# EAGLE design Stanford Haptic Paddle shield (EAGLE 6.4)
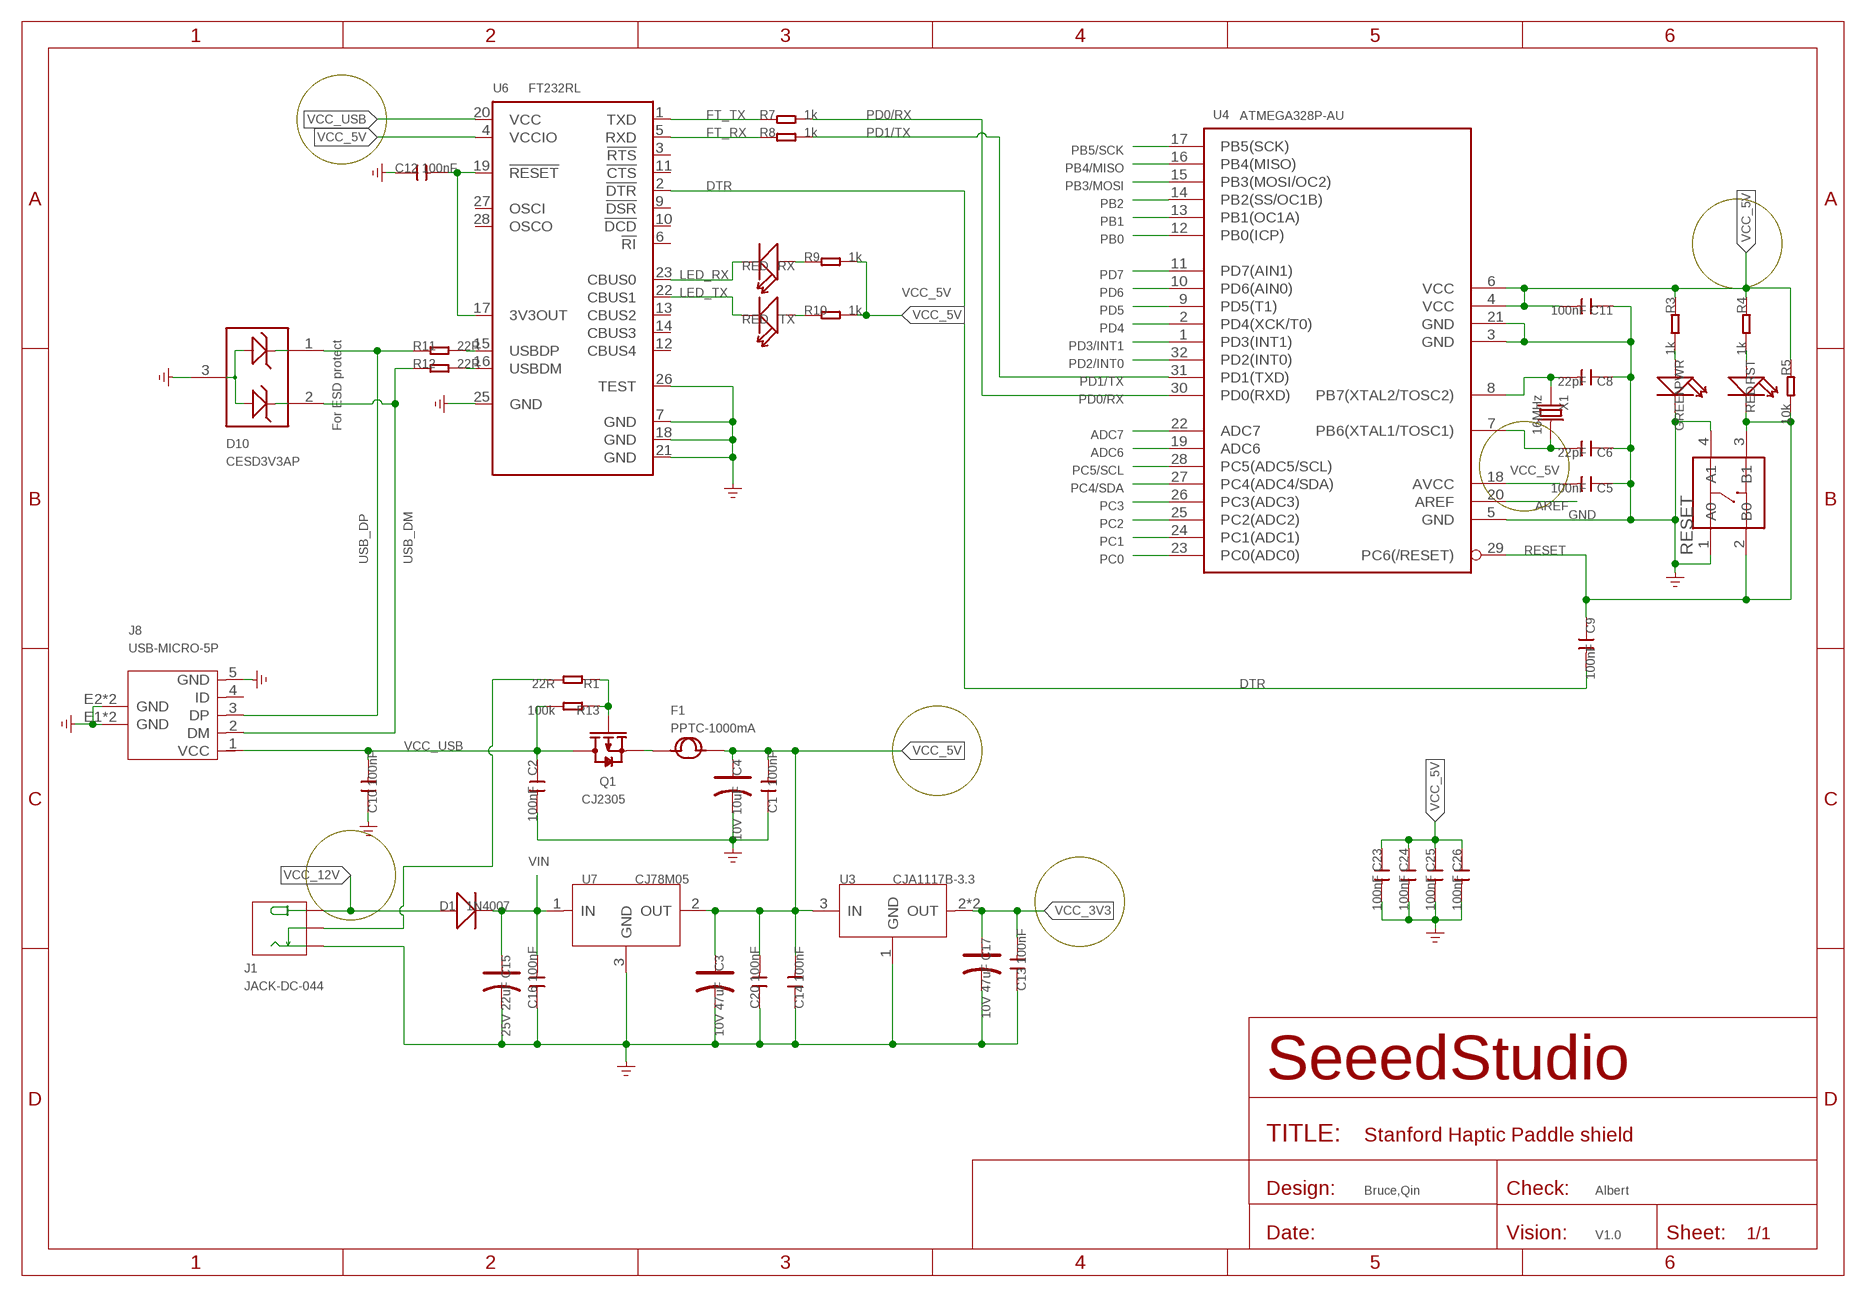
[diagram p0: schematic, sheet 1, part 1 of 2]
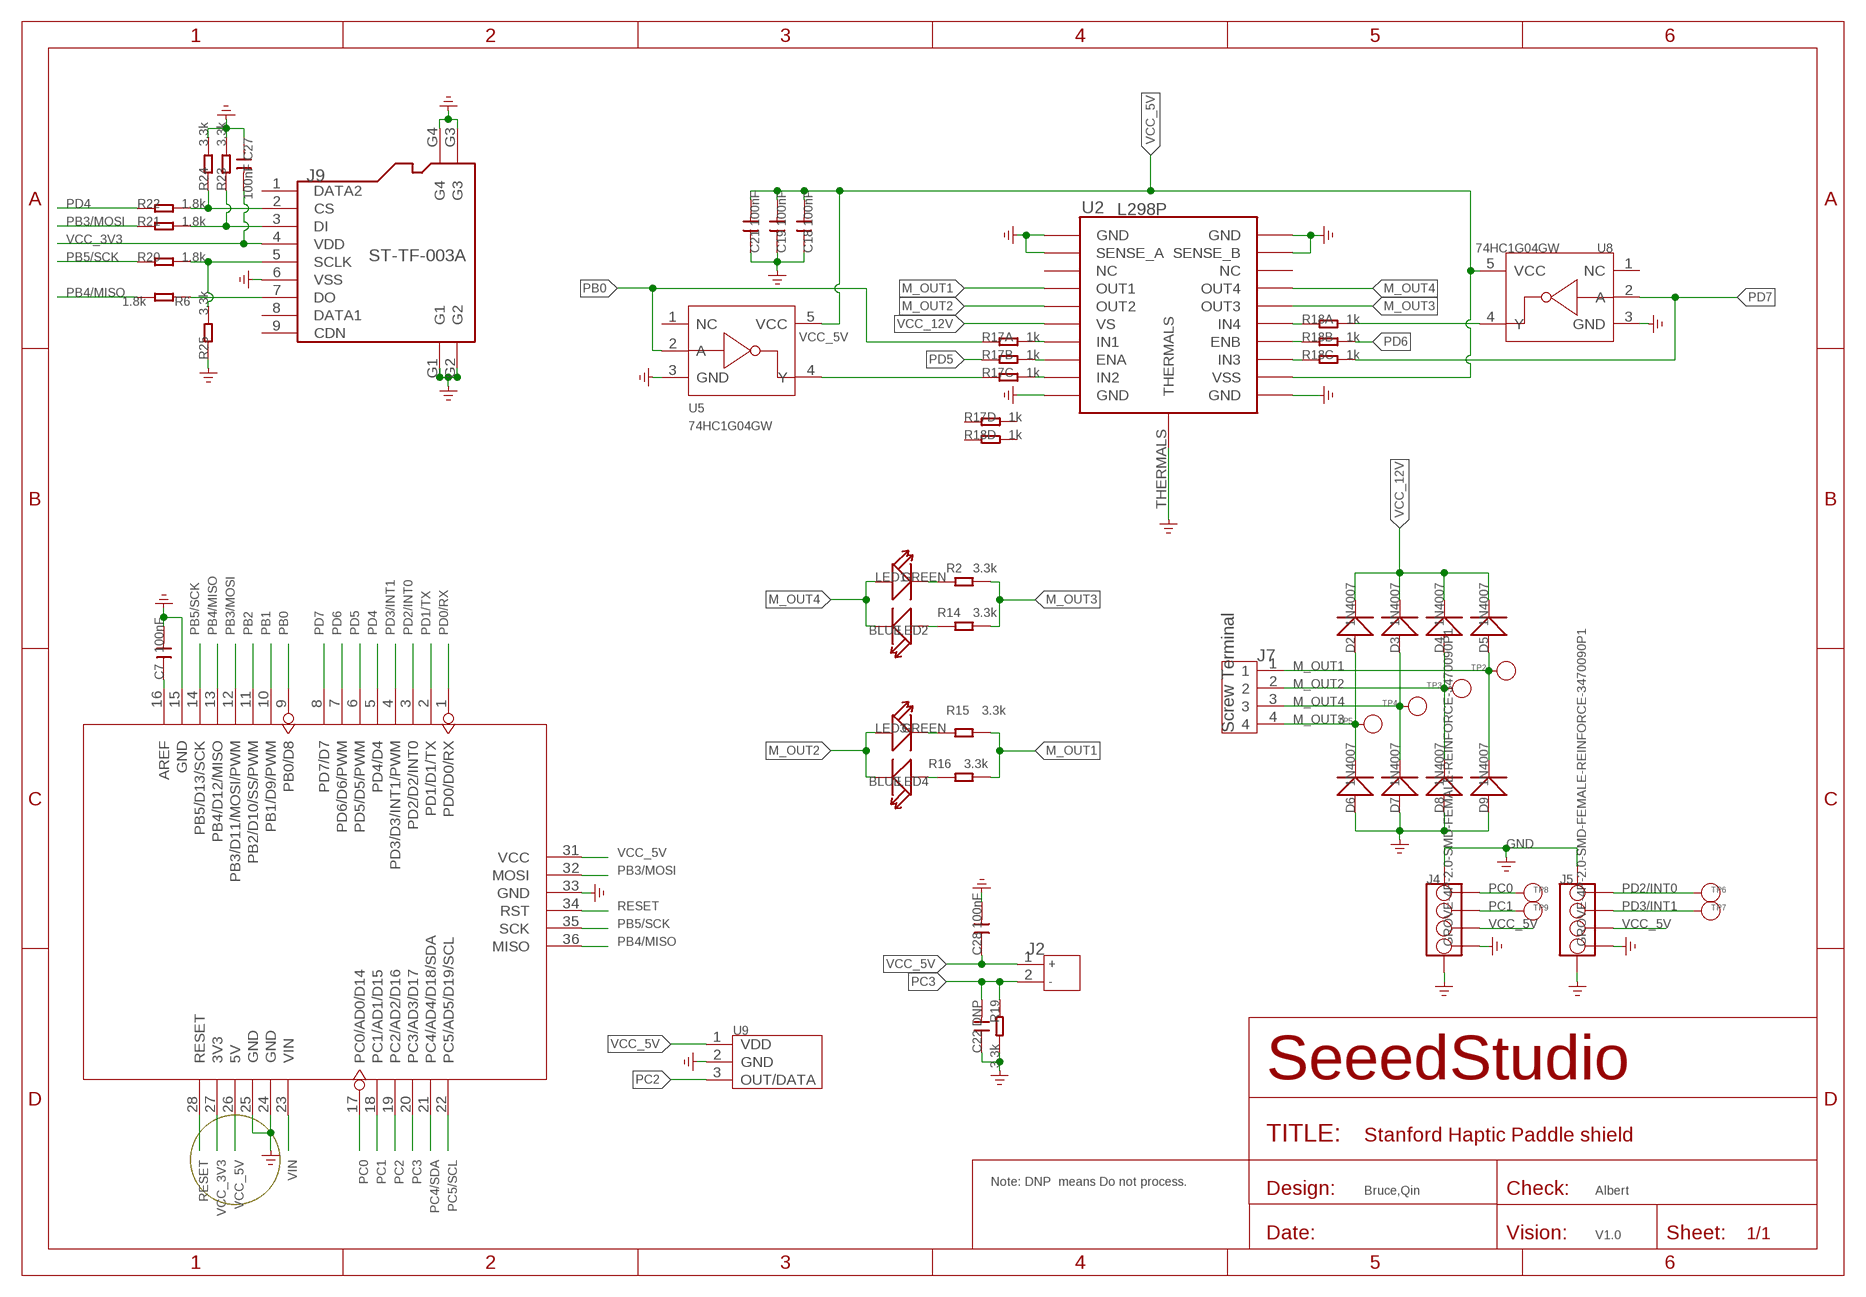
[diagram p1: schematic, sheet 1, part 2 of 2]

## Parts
C1  100nF  C-0603  [C0603]
C2  100nF  C-0603  [C0603]
C3  10V 47uF  CAP-AVX-B  [AVX-B]
C4  10V 10uF  C-POLAR-A  [AVX-A]
C5  100nF  C-0603  [C0603]
C6  22pF  C-0603  [C0603]
C7  100nF  C-0603  [C0603]
C8  22pF  C-0603  [C0603]
C9  100nF  C-0603  [C0603]
C10  100nF  C-0603  [C0603]
C11  100nF  C-0603  [C0603]
C12  100nF  C-0603  [C0603]
C13  100nF  C-0603  [C0603]
C14  100nF  C-0603  [C0603]
C15  25V 22uF  C-POLAR-C  [AVX-C]
C16  100nF  C-0603  [C0603]
C17  10V 47uF  CAP-AVX-B  [AVX-B]
C18  100nF  C-0603  [C0603]
C19  100nF  C-0603  [C0603]
C20  100nF  C-0603  [C0603]
C21  100nF  C-0603  [C0603]
C22  DNP  C-0603  [C0603]
C23  100nF  C-0603  [C0603]
C24  100nF  C-0603  [C0603]
C25  100nF  C-0603  [C0603]
C26  100nF  C-0603  [C0603]
C27  100nF  C-0603  [C0603]
C28  100nF  C-0603  [C0603]
D1  1N4007  D'B130L-13-F'  [SMA]
D2  1N4007  D'B130L-13-F'  [SMA]
D3  1N4007  D'B130L-13-F'  [SMA]
D4  1N4007  D'B130L-13-F'  [SMA]
D5  1N4007  D'B130L-13-F'  [SMA]
D6  1N4007  D'B130L-13-F'  [SMA]
D7  1N4007  D'B130L-13-F'  [SMA]
D8  1N4007  D'B130L-13-F'  [SMA]
D9  1N4007  D'B130L-13-F'  [SMA]
D10  CESD3V3AP  D-ESD-3P  [SOT23]
F1  PPTC-1000mA  FUSE'1206'  [F1206]
J1  JACK-DC-044  [DC-044]
J2  JACK-JST-2P-PW'2.0'  [JST-2.0]
J4  GROVE-4P-2.0-SMD-FEMALE-REINFORCE-3470090P1  [4P-SMD-2.0]
J5  GROVE-4P-2.0-SMD-FEMALE-REINFORCE-3470090P1  [4P-SMD-2.0]
J7  Screw Terminal  SCREW-TERMINAL-4P'3.5'  [4P-3.5]
J8  USB-MICRO-5P  [MICRO-USB-5P]
J9  ST-TF-003A  HOLDER-MICROSD-9P  [9P-SMD-W/-RING]
LED1  GREEN  LED'0603'  [LED-0603]
LED2  BLUE  LED'0603'  [LED-0603]
LED3  GREEN  LED'0603'  [LED-0603]
LED4  BLUE  LED'0603'  [LED-0603]
PWR  GREEN  LED'0603'  [LED-0603]
Q1  CJ2305  MOSFET-P'SI2323CDS/SI2305DS<BR>'  [SOT23]
R1  22R  R-0603  [R0603]
R2  3.3k  R-0603  [R0603]
R3  1k  R-0603  [R0603]
R4  1k  R-0603  [R0603]
R5  10k  R-0603  [R0603]
R6  1.8k  R-0603  [R0603]
R7  1k  R-0603  [R0603]
R8  1k  R-0603  [R0603]
R9  1k  R-0603  [R0603]
R10  1k  R-0603  [R0603]
R11  22R  R-0603  [R0603]
R12  22R  R-0603  [R0603]
R13  100k  R-0603  [R0603]
R14  3.3k  R-0603  [R0603]
R15  3.3k  R-0603  [R0603]
R16  3.3k  R-0603  [R0603]
R17  1k  R-4R-1206  [1206-8-3.3X2.4]
R18  1k  R-4R-1206  [1206-8-3.3X2.4]
R19  3.3k  R-0603  [R0603]
R20  1.8k  R-0603  [R0603]
R21  1.8k  R-0603  [R0603]
R22  1.8k  R-0603  [R0603]
R23  3.3k  R-0603  [R0603]
R24  3.3k  R-0603  [R0603]
R25  3.3k  R-0603  [R0603]
RESET  BUTTON-4P-6X6-SMD  [4P-SMD-6.2X6.2X4H]
RST  RED  LED'0603'  [LED-0603]
RX  RED  LED'0603'  [LED-0603]
TP2  PAD-TEST-POINT'3535'  [TP_3535]
TP3  PAD-TEST-POINT'3535'  [TP_3535]
TP4  PAD-TEST-POINT'3535'  [TP_3535]
TP5  PAD-TEST-POINT'3535'  [TP_3535]
TP6  PAD-TEST-POINT'3535'  [TP_3535]
TP7  PAD-TEST-POINT'3535'  [TP_3535]
TP8  PAD-TEST-POINT'3535'  [TP_3535]
TP9  PAD-TEST-POINT'3535'  [TP_3535]
TX  RED  LED'0603'  [LED-0603]
U1  ARDUINO'W/O-SILK'  [ARDUINO-W/O-SILK]
U2  L298P  [POWERSO-20]
U3  CJA1117B-3.3  CJ1117-3.3-1310120P1  [SOT89]
U4  ATMEGA328P-AU  ATMEGA8/168/328  [TQFP32]
U5  74HC1G04GW  74HC1G04  [SOT-353]
U6  FT232RL  [SSOP28]
U7  CJ78M05  78M05-TO252  [TO252]
U8  74HC1G04GW  74HC1G04  [SOT-353]
U9  SENSOR-MR-KMA210  [3P-5.55X1.55]
X1  16MHz  CRYSTAL'5032'  [2P-SMD-5X3.2]

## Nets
ADC6: U4.19(ADC6)
ADC7: U4.22(ADC7)
AREF: C7.1 U1.16(AREF) U4.20(AREF)
DTR: C9.2 U6.2(!DTR)
FT_RX: R8.1 U6.5(RXD)
FT_TX: R7.1 U6.1(TXD)
GATE: J1.CDN R1.2
GND: C1.1 C2.2 C3.- C4.- C5.1 C6.1 C7.2 C8.1 C10.1 C11.1 C12.1 C13.1 C14.1 C15.- C16.1 C17.- C18.1 C19.1 C20.1 C21.1 C22.1 C23.2 C24.2 C25.2 C26.2 C27.1 C28.2 D6.2(+) D7.2(+) D8.2(+) D9.2(+) D10.3 J1.- J4.4 J4.SS1 J4.SS2 J5.4 J5.SS1 J5.SS2 J8.5(GND) J8.E1(GND) J8.E2(GND) J8.P1(GND) J8.P2(GND) J9.6(VSS) J9.G1 J9.G2 J9.G3 J9.G4 PWR.- R19.2 R23.2 R24.2 R25.1 RESET.1(A0) RESET.4(A1) U1.15(GND) U1.24(GND) U1.25(GND) U1.33(GND) U2.P$1(GND) U2.P$2(SENSE_A) U2.P$10(GND) U2.P$11(GND) U2.P$19(SENSE_B) U2.P$20(GND) U2.THERMALS U3.1(GND) U4.3(GND) U4.5(GND) U4.21(GND) U5.3(GND) U6.7(GND) U6.18(GND) U6.21(GND) U6.25(GND) U6.26(TEST) U7.3(GND) U8.3(GND) U9.2(GND)
LED_RX: RX.- U6.23(CBUS0)
LED_TX: TX.- U6.22(CBUS1)
M_IN2: R17.3 U5.4(Y)
M_IN4: R18.8 U8.4(Y)
M_OUT1: D5.2(+) D9.1(-) J7.1 R15.1 R16.1 TP2.T U2.P$4(OUT1)
M_OUT2: D4.2(+) D8.1(-) J7.2 LED3.+ LED4.- TP3.T U2.P$5(OUT2)
M_OUT3: D2.2(+) D6.1(-) J7.4 R2.1 R14.1 TP5.T U2.P$16(OUT3)
M_OUT4: D3.2(+) D7.1(-) J7.3 LED1.+ LED2.- TP4.T U2.P$17(OUT4)
N$1: Q1.1(G) R1.1 R13.1
N$2: R12.2 U6.16(USBDM)
N$3: J9.7(DO) R6.1
N$4: R11.2 U6.15(USBDP)
N$5: LED1.- R2.2
N$6: C12.2 U6.17(3V3OUT) U6.19(!RESET)
N$7: PWR.+ R3.2
N$8: LED2.+ R14.2
N$9: LED3.- R15.2
N$10: LED4.+ R16.2
N$11: J9.5(SCLK) R20.2 R25.2
N$12: J9.3(DI) R21.2 R23.1
N$13: J9.2(CS) R22.2 R24.1
N$14: R17.8 U2.P$7(IN1)
N$15: R17.7 U2.P$8(ENA)
N$16: R17.6 U2.P$9(IN2)
N$17: R4.2 RST.+
N$21: R18.3 U2.P$13(IN3)
N$22: R18.2 U2.P$14(ENB)
N$23: R18.1 U2.P$15(IN4)
N$31: R9.1 RX.+
N$32: R10.1 TX.+
P5V: F1.1 Q1.2(S)
PB0: R17.1 U1.9(PB0/D8) U4.12(PB0(ICP)) U5.2(A)
PB1: U1.10(PB1/D9/PWM) U4.13(PB1(OC1A))
PB2: U1.11(PB2/D10/SS/PWM) U4.14(PB2(SS/OC1B))
PB3/MOSI: R21.1 U1.12(PB3/D11/MOSI/PWM) U1.32(MOSI) U4.15(PB3(MOSI/OC2))
PB4/MISO: R6.2 U1.13(PB4/D12/MISO) U1.36(MISO) U4.16(PB4(MISO))
PB5/SCK: R20.1 U1.14(PB5/D13/SCK) U1.35(SCK) U4.17(PB5(SCK))
PC0: J4.1 TP8.T U1.17(PC0/AD0/D14) U4.23(PC0(ADC0))
PC1: J4.2 TP9.T U1.18(PC1/AD1/D15) U4.24(PC1(ADC1))
PC2: U1.19(PC2/AD2/D16) U4.25(PC2(ADC2)) U9.3(OUT/DATA)
PC3: C22.2 J2.2 R19.1 U1.20(PC3/AD3/D17) U4.26(PC3(ADC3))
PC4/SDA: U1.21(PC4/AD4/D18/SDA) U4.27(PC4(ADC4/SDA))
PC5/SCL: U1.22(PC5/AD5/D19/SCL) U4.28(PC5(ADC5/SCL))
PD0/RX: R7.2 U1.1(PD0/D0/RX) U4.30(PD0(RXD))
PD1/TX: R8.2 U1.2(PD1/D1/TX) U4.31(PD1(TXD))
PD2/INT0: J5.1 TP6.T U1.3(PD2/D2/INT0) U4.32(PD2(INT0))
PD3/INT1: J5.2 TP7.T U1.4(PD3/D3/INT1/PWM) U4.1(PD3(INT1))
PD4: R22.1 U1.5(PD4/D4) U4.2(PD4(XCK/T0))
PD5: R17.2 U1.6(PD5/D5/PWM) U4.9(PD5(T1))
PD6: R18.7 U1.7(PD6/D6/PWM) U4.10(PD6(AIN0))
PD7: R18.6 U1.8(PD7/D7) U4.11(PD7(AIN1)) U8.2(A)
RESET: C9.1 R5.2 RESET.2(B0) RESET.3(B1) RST.- U1.28(RESET) U1.34(RST) U4.29(PC6(/RESET))
USB_DM: D10.2 J8.2(DM) R12.1
USB_DP: D10.1 J8.3(DP) R11.1
VCC_3V3: C13.2 C17.+ C27.2 J9.4(VDD) U1.27(3V3) U3.2(OUT) U3.4(OUT)
VCC_5V: C1.2 C3.+ C4.+ C5.2 C11.2 C14.2 C18.2 C19.2 C20.2 C21.2 C23.1 C24.1 C25.1 C26.1 C28.1 F1.2 J2.1 J4.3 J5.3 R3.1 R4.1 R5.1 R9.2 R10.2 U1.26(5V) U1.31(VCC) U2.P$12(VSS) U3.3(IN) U4.4(VCC) U4.6(VCC) U4.18(AVCC) U5.5(VCC) U6.4(VCCIO) U7.2(OUT) U8.5(VCC) U9.1(VDD)
VCC_12V: D1.2(+) D2.1(-) D3.1(-) D4.1(-) D5.1(-) J1.+ U2.P$6(VS)
VCC_USB: C2.1 C10.2 J8.1(VCC) Q1.3(D) R13.2 U6.20(VCC)
VIN: C15.+ C16.2 D1.1(-) U1.23(VIN) U7.1(IN)
XTAL1: C6.2 U4.7(PB6(XTAL1/TOSC1)) X1.2
XTAL2: C8.2 U4.8(PB7(XTAL2/TOSC2)) X1.1
Unconnected: J8.4(ID) J9.1(DATA2) J9.8(DATA1) J9.9(CDN) R17.4 R17.5 R18.4 R18.5 U2.P$3(NC) U2.P$18(NC) U5.1(NC) U6.3(!RTS) U6.6(!RI) U6.9(!DSR) U6.10(!DCD) U6.11(!CTS) U6.12(CBUS4) U6.13(CBUS2) U6.14(CBUS3) U6.27(OSCI) U6.28(OSCO) U8.1(NC)

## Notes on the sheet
- For ESD protect
- Note: DNP  means Do not process.
- Bruce,Qin | Albert | Bruce,Qin | Albert
- V1.0 | V1.0

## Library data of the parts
C1 C2 C5-C14 C16 C18-C28 = Discrete:C*: Ceramic Capacitors
C3 C17 = Discrete:CAP*: Electrolytic Capacitors,Tantalum Capacitors and Super Capacitors
C4 C15 = OPL:C-POLAR*
D1-D9 = Discrete:D*
D10 = Discrete:D-ESD-3P
F1 = Discrete:FUSE
J1 = Connector :JACK-DC-044
J2 = Connector :JACK-JST-2P-PW
J4 J5 = OPL:GROVE-4P-2.0-SMD-FEMALE-REINFORCE
J7 = Connector :SCREW-TERMINAL-4P
J8 = Connector :USB-MICRO-5P
J9 = Connector :HOLDER-MICROSD-9P
LED1-LED4 PWR RST RX TX = Discrete:LED*
Q1 = Discrete:MOSFET-P
R1-R16 R19-R25 = Discrete:R*
R17 R18 = Discrete:R-4R*: Resistor Array
RESET = Discrete:BUTTON-4P
TP2-TP9 = Discrete:PAD-TEST-POINT; PARTNO: DNP
U1 = moudle:ARDUINO
U2 = IC:L298: Dual Full-Bridge Driver http://www.sandorobotics.com/attachments/l298motores.pdf
U3 = OPL:CJ1117-3.3: 1A Low Dropout Linear Regulator
U4 = IC:ATMEGA8/168/328: MICROCONTROLLER
U5 U8 = template:74HC1G04: 74HC1G04 and 74HCT1G04 are high-speed Si-gate CMOS devices. They provide an inverting buffer.
U6 = IC_SMD:FT232R: Source: http://www.ftdichip.com/Documents/DataSheets/DS_FT232R_v104.pdf
U7 = IC:78M05: 0.5A Three Terminal Positive Voltage Regulators
U9 = template:SENSOR-MR
X1 = Discrete:CRYSTAL*: CRYSTAL

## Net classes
0 default: clearance 0.152 mm
3 usbvcc: width 0.203 mm, drill 0.305 mm, clearance 0.203 mm

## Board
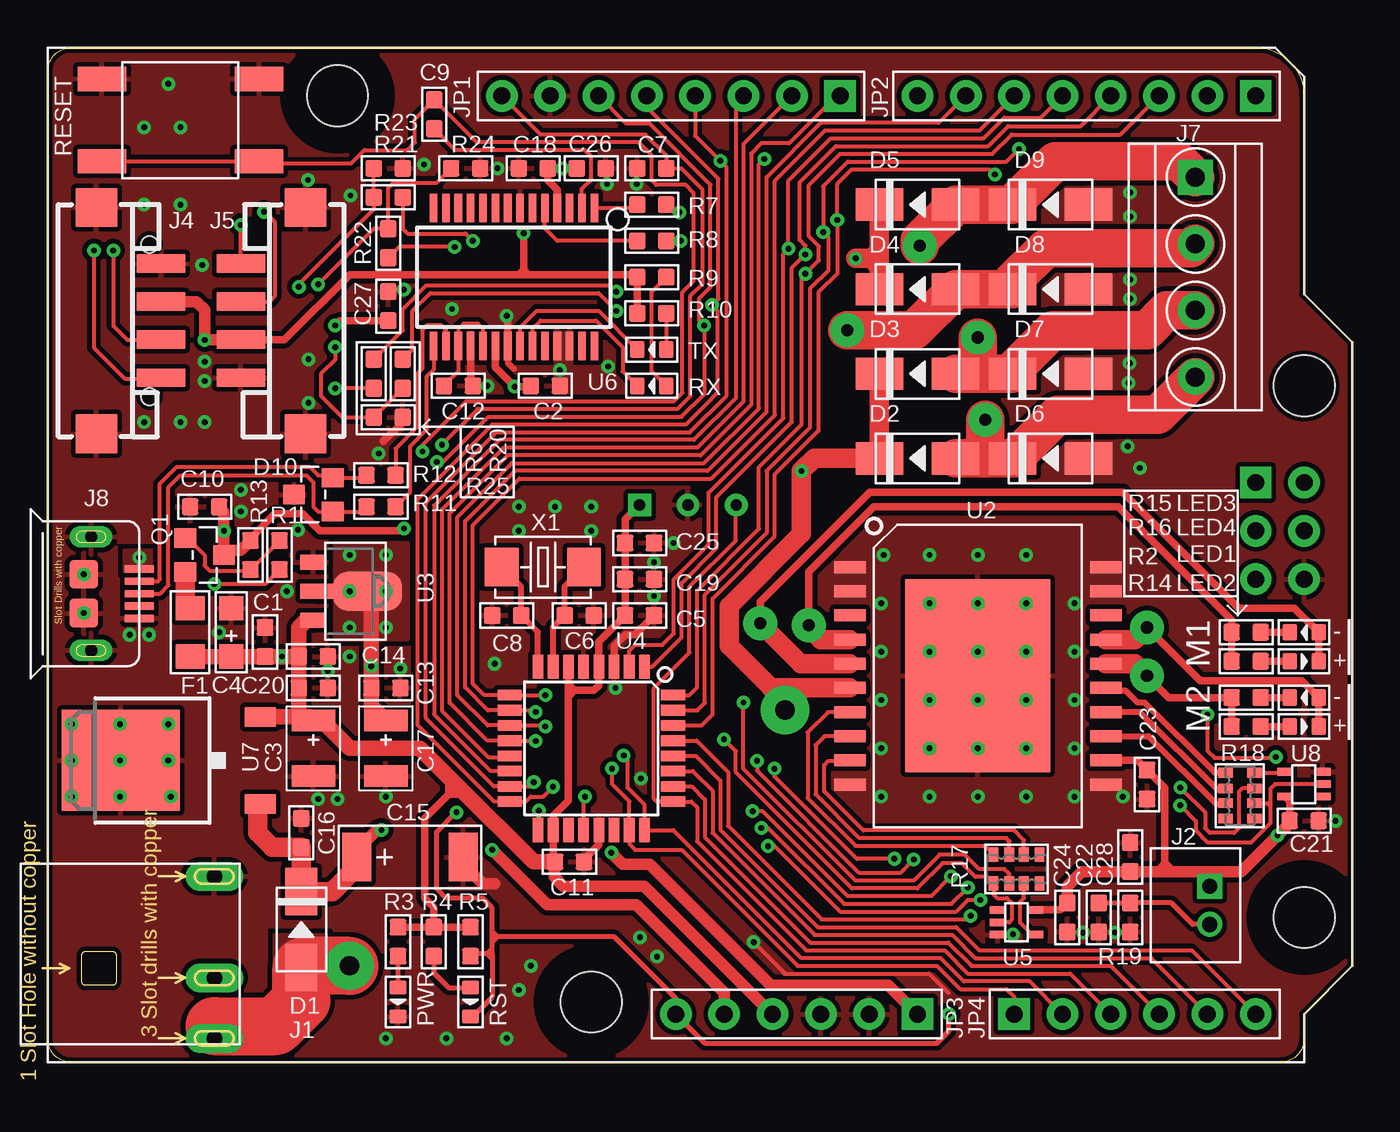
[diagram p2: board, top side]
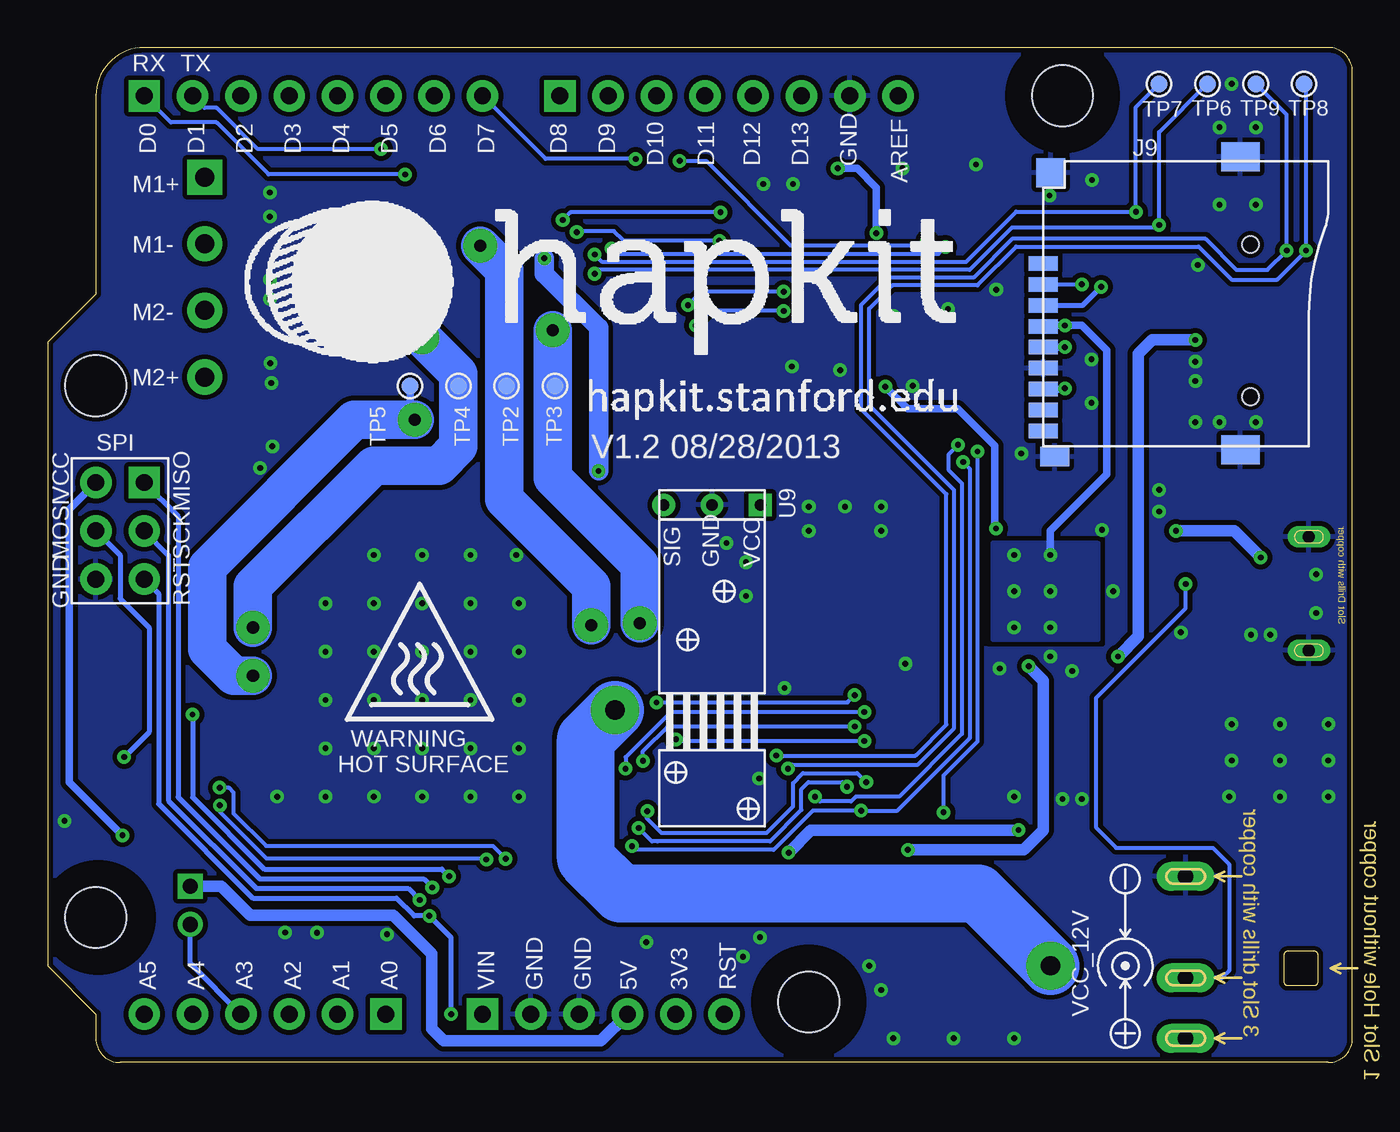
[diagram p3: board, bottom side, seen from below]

Size 68.58 x 53.34 mm. Coordinates in mm from the lower left corner, seen from the top.
Outline: 66.04,2.54 66.04,1.27 arc-90 64.77,0 1.27,0 arc-90 0,1.27 0,52.07 arc-90 1.27,53.34 63.5,53.34 arc-90 66.04,50.8 66.04,40.39 68.58,37.85 68.58,5.08 66.04,2.54
Copper layers (1*16): Top 0.035mm / dielectric 1.5mm / Bottom 0.035mm
Design rules "default *": minimum track width 8mil, minimum drill 12mil, track to track 8mil, track to pad 8mil, pad to pad 8mil, via to via 8mil, smd to smd 0mil, copper to edge 10mil, drill to drill 8mil, minimum pad ring 10mil, minimum via ring 8mil, stop-mask expansion 4mil, vias tented up to drill 100mil, thermal gap 10mil
Holes 3.2 mm at 28.57,3.17
tRestrict: area -68.6,-23.4 to -68.5,-23.2; area 12.5,48 to 18,53.5; area 63.3,4.9 to 68.8,10.4; area 25.8,0.4 to 31.3,5.9
bRestrict: area 12.5,48 to 18,53.5; area 63.2,4.9 to 68.7,10.4; area 25.8,0.4 to 31.3,5.9

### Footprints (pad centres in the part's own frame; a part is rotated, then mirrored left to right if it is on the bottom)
C0603 = smd 0.889 x 0.889: 1 -0.762,0; 2 0.762,0
AVX-B = smd 1.143 x 2.286: + -1.46,0; - 1.46,0
AVX-A = smd 1.27 x 1.27: + -1.27,0; - 1.27,0
AVX-C = smd 1.524 x 2.54: + -2.794,0; - 2.794,0
SMA = smd 2.5 x 1.7: 1 2,0; 2 -2,0
SOT23 = smd 1.016 x 1.143: 1 -0.889,-1.016; 2 0.889,-1.016; 3 0,1.016
F1206 = smd 1.27 x 1.524: 1 -1.27,0; 2 1.27,0
DC-044 = drill 0.813 pad 1.524 long: + 3.175,10.16; - -5.334,10.16; CDN 0,10.16
JST-2.0 = drill 0.8 pad 1.3 square: 1 -1,0.75 | drill 0.8 pad 1.3: 2 1,0.75
4P-SMD-2.0 = smd 0.965 x 2.54: 1 -3,0; 2 -1,0; 3 1,0; 4 3,0 | smd 2.032 x 2.184: SS1 -5.946,3.4; SS2 5.946,3.4
4P-3.5 = drill 1 pad 1.85 square: 1 -5.25,0 | drill 1 pad 1.85: 2 -1.75,0; 3 1.75,0; 4 5.25,0
MICRO-USB-5P = smd 0.38 x 1.52: 1 -1.3,0; 2 -0.65,0; 3 0,0; 4 0.65,0; 5 1.3,0 | smd 1.524 x 1.524: E1 -1.016,-2.921; E2 1.016,-2.921 | drill 0.635 pad 1.143 long: P1 -2.985,-2.54; P2 2.985,-2.54
9P-SMD-W/-RING = smd 1.524 x 0.762: 1 0,4.4; 2 0,3.3; 3 0,2.2; 4 0,1.1; 5 0,0; 6 0,-1.1; 7 0,-2.2; 8 0,-3.3; 9 0,-4.4 | smd 1.524 x 1.016: G1 0.6,-5.746 | smd 2.032 x 1.524: G2 10.373,-5.4; G3 10.373,10 | smd 1.524 x 1.524: G4 0.392,9.181 | hole 0.889: 10.9,-2.6; 10.9,5.4
LED-0603 = smd 0.762 x 0.889: + -0.762,0; - 0.762,0
R0603 = smd 0.889 x 0.889: 1 -0.762,0; 2 0.762,0
1206-8-3.3X2.4 = smd 0.508 x 0.762: 1 -1.206,-0.762; 2 -0.381,-0.762; 3 0.381,-0.762; 4 1.206,-0.762; 5 1.206,0.762; 6 0.381,0.762; 7 -0.381,0.762; 8 -1.206,0.762
4P-SMD-6.2X6.2X4H = smd 2.54 x 1.27: 1 -4.129,2.159; 2 -4.129,-2.159; 3 4.129,-2.159; 4 4.129,2.159
TP_3535 = smd 0.889 x 0.889: T 0,0
ARDUINO-W/O-SILK = drill 0.889 pad 1.651 square: 1 63.5,50.8; 9 41.656,50.8; 17 50.8,2.54; 23 45.72,2.54; 36 63.5,30.48 | drill 0.889 pad 1.651: 2 60.96,50.8; 3 58.42,50.8; 4 55.88,50.8; 5 53.34,50.8; 6 50.8,50.8; 7 48.26,50.8; 8 45.72,50.8; 10 39.116,50.8; 11 36.576,50.8; 12 34.036,50.8; 13 31.496,50.8; 14 28.956,50.8; 15 26.416,50.8; 16 23.876,50.8; 18 53.34,2.54; 19 55.88,2.54; 20 58.42,2.54; 21 60.96,2.54; 22 63.5,2.54; 24 43.18,2.54; 25 40.64,2.54; 26 38.1,2.54; 27 35.56,2.54; 28 33.02,2.54; 31 66.04,30.48; 32 66.04,27.94; 33 66.04,25.4; 34 63.5,25.4; 35 63.5,27.94 | hole 3.2: 15.24,50.8; 66.04,35.56; 66.04,7.62
POWERSO-20 = smd 1.651 x 0.635: P$1 -6.731,5.715; P$2 -6.731,4.445; P$3 -6.731,3.175; P$4 -6.731,1.905; P$5 -6.731,0.635; P$6 -6.731,-0.635; P$7 -6.731,-1.905; P$8 -6.731,-3.175; P$9 -6.731,-4.445; P$10 -6.731,-5.715; P$11 6.731,-5.715; P$12 6.731,-4.445; P$13 6.731,-3.175; P$14 6.731,-1.905; P$15 6.731,-0.635; P$16 6.731,0.635; P$17 6.731,1.905; P$18 6.731,3.175; P$19 6.731,4.445; P$20 6.731,5.715 | smd 7.62 x 10.16: THERMALS 0,0
SOT89 = smd 0.8 x 1.4: 1 -1.524,-1.905; 3 1.524,-1.905 | smd 0.8 x 1.9: 2 0,-1.651 | smd 2.032 x 3.65: 4 0,0.94
TQFP32 = smd 1.27 x 0.559: 1 -4.293,2.8; 2 -4.293,2; 3 -4.293,1.2; 4 -4.293,0.4; 5 -4.293,-0.4; 6 -4.293,-1.2; 7 -4.293,-2; 8 -4.293,-2.8; 17 4.293,-2.8; 18 4.293,-2; 19 4.293,-1.2; 20 4.293,-0.4; 21 4.293,0.4; 22 4.293,1.2; 23 4.293,2; 24 4.293,2.8 | smd 0.559 x 1.27: 9 -2.8,-4.293; 10 -2,-4.293; 11 -1.2,-4.293; 12 -0.4,-4.293; 13 0.4,-4.293; 14 1.2,-4.293; 15 2,-4.293; 16 2.8,-4.293; 25 2.8,4.293; 26 2,4.293; 27 1.2,4.293; 28 0.4,4.293; 29 -0.4,4.293; 30 -1.2,4.293; 31 -2,4.293; 32 -2.8,4.293
SOT-353 = smd 0.4 x 0.8: 1 -0.65,-1; 2 0,-1; 3 0.65,-1; 4 0.65,1; 5 -0.65,1
SSOP28 = smd 0.4 x 1.5: 1 -4.225,-3.625; 2 -3.575,-3.625; 3 -2.925,-3.625; 4 -2.275,-3.625; 5 -1.625,-3.625; 6 -0.975,-3.625; 7 -0.325,-3.625; 8 0.325,-3.625; 9 0.975,-3.625; 10 1.625,-3.625; 11 2.275,-3.625; 12 2.925,-3.625; 13 3.575,-3.625; 14 4.225,-3.625; 15 4.225,3.625; 16 3.575,3.625; 17 2.925,3.625; 18 2.275,3.625; 19 1.625,3.625; 20 0.975,3.625; 21 0.325,3.625; 22 -0.325,3.625; 23 -0.975,3.625; 24 -1.625,3.625; 25 -2.275,3.625; 26 -2.925,3.625; 27 -3.575,3.625; 28 -4.225,3.625
TO252 = smd 1.016 x 1.651: 1 -2.286,-4.826; 2 2.286,-4.826 | smd 5.3 x 6.2: 3 0,2.5
3P-5.55X1.55 = drill 0.6 pad 1.2 square: 1 -2.54,0 | drill 0.6 pad 1.2: 2 0,0; 3 2.54,0
2P-SMD-5X3.2 = smd 1.778 x 2.032: 1 -2.159,0; 2 2.159,0

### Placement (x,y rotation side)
C1  11.43,22.1 270 top
C2  26.16,35.56 0 top
C3  13.97,16.51 270 top
C4  9.65,22.61 90 top
C5  31.11,23.5 180 top
C6  27.94,23.5 180 top
C7  31.75,46.99 180 top
C8  24.13,23.5 0 top
C9  20.32,49.83 270 top
C10  8.26,29.21 0 top
C11  27.43,10.54 180 top
C12  21.59,35.56 180 top
C13  17.78,19.68 180 top
C14  13.97,21.34 180 top
C15  19.05,10.79 0 top
C16  13.34,12.06 270 top
C17  17.78,16.51 270 top
C18  25.53,46.99 0 top
C19  31.11,25.4 180 top
C20  13.97,19.68 180 top
C21  66.04,12.7 180 top
C22  55.24,7.62 90 top
C23  57.78,14.61 270 top
C24  53.59,7.62 270 top
C25  31.11,27.3 0 top
C26  28.57,46.99 0 top
C27  17.91,39.75 270 top
C28  56.9,10.79 90 top
D1  13.34,6.99 90 top
D2  45.72,31.75 180 top
D3  45.72,36.2 180 top
D4  45.72,40.64 180 top
D5  45.72,45.09 180 top
D6  52.7,31.75 180 top
D7  52.7,36.2 180 top
D8  52.7,40.64 180 top
D9  52.7,45.09 180 top
D10  13.97,29.84 90 top
F1  7.49,22.61 270 top
J1  -1.4,4.45 270 top
J2  60.33,8.26 270 top
J4  5.97,38.99 90 top
J5  10.16,38.99 270 top
J7  60.33,41.27 270 top
J8  4.83,24.64 270 top
J9  16.26,37.59 0 bottom
LED1  66.04,19.18 180 top
LED2  66.04,17.65 0 top
LED3  66.04,22.61 180 top
LED4  66.04,21.08 0 top
PWR  18.41,3.17 270 top
Q1  8.26,26.67 270 top
R1  12.19,26.67 270 top
R2  62.99,19.18 0 top
R3  18.41,6.35 270 top
R4  20.29,6.35 270 top
R5  22.23,6.35 270 top
R6  17.14,36.2 90 top
R7  31.75,45.09 0 top
R8  31.75,43.18 0 top
R9  31.75,41.27 180 top
R10  31.75,39.37 180 top
R11  17.53,29.21 0 top
R12  17.53,30.86 0 top
R13  10.67,26.67 90 top
R14  62.99,17.65 0 top
R15  62.99,22.61 0 top
R16  62.99,21.08 0 top
R17  50.93,10.16 0 top
R18  62.66,14.02 270 top
R19  56.9,7.62 270 top
R20  18.67,36.2 270 top
R21  17.91,45.47 180 top
R22  17.91,43.05 90 top
R23  17.91,46.99 0 top
R24  21.97,46.99 0 top
R25  17.91,33.91 180 top
RESET  6.99,49.53 0 top
RST  22.23,3.17 270 top
RX  31.75,35.56 180 top
TP2  44.45,35.56 270 bottom
TP3  41.91,35.56 270 bottom
TP4  46.99,35.56 270 bottom
TP5  49.53,35.56 270 bottom
TP6  7.62,51.44 90 bottom
TP7  10.16,51.44 90 bottom
TP8  2.54,51.44 90 bottom
TP9  5.08,51.44 90 bottom
TX  31.75,37.47 180 top
U1  0,0 0 top
U2  48.9,20.32 0 top
U3  15.88,24.77 270 top
U4  28.57,16.51 270 top
U5  50.93,7.37 270 top
U6  24.51,41.27 180 top
U7  6.35,15.88 90 top
U8  66.03,14.63 90 top
U9  33.66,29.3 180 bottom
X1  26.04,26.04 0 top

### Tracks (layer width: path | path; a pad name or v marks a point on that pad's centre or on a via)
AREF  (via drill 0.3 pad 0.64)
  Top 0.203: v20.73,32.46 22.61,34.34 33.11,34.34 33.79,35.02 33.79,40.29 34.41,40.91 34.41,45.9 33.31,46.99 C7.1 32.51,47.67 31.41,48.77 25.91,48.77 U1.16 | U4.20 28.18,13.9 v28.25,13.97
  Bottom 0.203: v20.73,32.46 21.21,31.98 21.21,31.11 20.52,30.43 20.52,17.27 23.82,13.97 26.1,13.97 26.35,13.72 27.99,13.72 v28.25,13.97
DTR
  Top 0.203: U6.2 28.09,45.91 28.57,46.4 28.57,47.62 28.25,47.95 21.44,47.95 C9.2
FT_RX
  Top 0.203: R8.1 26.79,43.18 26.14,43.84 U6.5
FT_TX
  Top 0.203: 30.8,44.9 U6.1
  Top 0.254: 30.8,44.9 R7.1
GATE  (via drill 0.3 pad 0.64)
  Top 0.203: R1.2 11.43,25.15 v8.76,25.15
  Bottom 0.203: J1.CDN 6.86,4.45 6.48,4.83 6.48,10.41 7.34,11.28 12.42,11.28 13.46,12.32 13.46,19.18 8.76,23.88 v8.76,25.15
GND  (via drill 0.3 pad 0.64)
  Top 0.203: 47.35,3.66 46.33,4.67 38.7,4.67 38.7,4.74 37.08,6.35
  Top 0.254: U5.3 50.05,6.72
  Top 0.305: U6.21 24.19,36.77 24.51,36.45
  Top 0.406: U4.3 29.77,21.9 30.35,22.48 30.86,22.48 C5.1 | U4.21 28.98,11.45 28.19,10.67 C11.1 | R25.1 18.67,33.66 17.65,32.64 | U6.21 24.19,39.19 v24.13,39.24 | U6.18 22.24,35.68 C12.1
  Top 0.61: C15.- 21.84,10.41 22.86,9.4 23.5,9.4
  other vias: 56.82,35.71 56.87,36.75 57.4,31.24 56.77,32.38 56.9,41.15 56.9,40.13 56.9,45.72 56.9,44.45 50.74,6.73 54.42,6.82 56.1,6.83 23.11,35.56 26.92,36.39 29.46,36.58 1.27,17.78 3.81,17.78 6.35,17.78 6.35,15.88 3.81,15.88 1.27,15.88 3.81,13.97 6.48,13.97 1.27,13.97 46.35,24.13 48.9,24.13 51.44,24.13 51.44,21.59 48.9,21.59 46.35,21.59 46.35,19.05 48.9,19.05 51.44,19.05 51.44,26.67 48.9,16.51 46.35,16.51 5.33,22.48 9.02,22.61 12.57,24.77 10.16,30.1 10.16,28.96 13.16,27.99 15.88,21.34 18.54,20.7 14.73,20.57 15.24,13.84 14.22,13.84 17.78,13.97 24.77,3.81 23.5,20.95 24.77,27.94 32.89,27.3 31.88,24.51 31.88,26.29 8.26,33.66 8.26,36.83 29.4,46.16 24.77,29.21 26.67,29.21 28.57,29.21 28.57,27.94 13.72,34.67 13.72,36.96 5.08,33.66 6.99,33.66 46.35,26.67 48.9,26.67 46.35,13.97 48.9,13.97 51.44,13.97 53.98,13.97 53.98,16.51 53.98,19.05 53.98,21.59 53.98,24.13 43.81,24.13 43.81,21.59 43.81,19.05 43.81,16.51 43.81,13.97 43.94,26.67 51.44,16.51 37.11,6.32 23.65,46.99 19.79,47.19 13.69,46.38 15.93,45.57 30.96,46.16 21.26,39.6 18.72,40.61 31.18,14.92 29.84,19.68 1.91,23.62 1.91,25.65 5.08,45.09 6.99,45.09 5.08,49.15 6.99,49.15 6.35,51.44 8.13,41.91 8.26,35.81 17.4,32 4.32,22.48 24.13,1.27 20.95,1.27 17.78,1.27 56.52,13.97 67.69,12.7 25.4,5.08 31.14,6.58 32.03,5.56
  pour Top (isolate 0.254, rank 6): 0,53.34 68.58,53.34 68.58,0 0,0
  pour Bottom (isolate 0.254, rank 6): 0,53.34 68.58,53.34 68.58,0 0,0
  pour Top (isolate 0.254, no thermals): 40.64,24.13 43.81,24.13 43.81,26.67 40.64,26.67
  pour Top (isolate 0.254, no thermals): 53.98,24.13 57.15,24.13 57.15,26.67 53.98,26.67
  pour Top (isolate 0.254, no thermals): 54.61,13.97 56.9,13.97 56.9,15.24 54.61,15.24
  pour Top (isolate 0.254, no thermals): 41.27,13.97 43.18,13.97 43.18,15.24 41.27,15.24
  pour Top (isolate 0.254, no thermals): 27.56,35.18 27.56,38.35 26.67,38.35 26.67,35.18
  pour Top (isolate 0.254, no thermals): 53.09,32.89 57.78,32.89 57.78,30.48 53.09,30.48
  pour Top (isolate 0.254, no thermals): 52.45,37.34 57.15,37.34 57.15,34.92 52.45,34.92
  pour Top (isolate 0.254, no thermals): 52.45,41.78 57.15,41.78 57.15,39.37 52.45,39.37
  pour Top (isolate 0.254, no thermals): 52.45,46.23 57.15,46.23 57.15,43.81 52.45,43.81
LED_RX
  Top 0.203: RX.- 30.23,36.32 30.23,37.59 28.83,38.99 25.91,38.99 25.49,38.57 U6.23
LED_TX
  Top 0.203: 30.73,37.47 TX.- | U6.22 24.83,37.66 24.83,38.61 25.72,39.5 28.96,39.5 TX.- | 30.86,37.47 TX.-
M_IN2
  Top 0.203: U5.4 51.75,6.72 51.12,7.35 51.12,8.44 51.31,8.64 R17.3
M_IN4
  Top 0.203: R18.8 64.97,15.23 U8.4
M_OUT1  (via drill 0.64 pad 1.78)
  Top 0.406: v40.01,22.99 40.01,25.79 43.42,29.21 56.26,29.21 62.23,23.24 R15.1 R16.1
  Top 1.016: U2.P$4 40.64,22.23 40.01,22.86 v40.01,22.99
  Top 2.032: v45.85,42.93 45.85,43.21 D5.2 D9.1 50.7,45.12 52.96,47.37 59.48,47.37 J7.1
  Bottom 0.406: TP2.T 44.45,41.53 v45.85,42.93
  Bottom 2.032: v40.01,22.99 40.01,25.02 44.58,29.59 44.58,41.66 v45.85,42.93
M_OUT2  (via drill 0.64 pad 1.78)
  Top 0.406: v37.47,23.08 37.47,24.22 43.22,29.97 56.52,29.97 62.61,23.88 65.53,23.88 LED3.+ LED4.-
  Top 1.016: U2.P$5 39.59,20.95 v37.47,23.08
  Top 2.032: v42.04,38.48 45.56,38.48 D4.2 D8.1 50.7,41.05 52.45,42.8 60.1,42.8 J7.2
  Bottom 0.406: v42.04,38.48 42.04,35.69 TP3.T
  Bottom 2.032: v42.04,38.48 42.04,30.73 37.47,26.16 v37.47,23.08
M_OUT3  (via drill 0.64 pad 1.78)
  Top 0.406: R14.1 R2.1 58.93,19.18 v57.78,20.32
  Top 1.016: U2.P$16 57.15,20.95 v57.78,20.32
  Top 2.032: 49.4,31.75 D6.1 50.8,31.75 53.09,34.04 58.34,34.04 J7.4 | 49.4,31.75 D2.2 | v49.28,33.78 49.28,31.88 49.4,31.75
  Bottom 0.406: TP5.T 49.53,33.78
  Bottom 2.032: v57.78,20.32 58.8,20.32 60.2,21.72 60.2,26.04 52.45,33.78 49.53,33.78 v49.28,33.78
M_OUT4  (via drill 0.64 pad 1.78)
  Top 0.406: LED2.- LED1.+ 65.91,20.07 60.58,20.07 v57.78,22.86
  Top 1.016: U2.P$17 57.15,22.23 v57.78,22.86
  Top 2.032: v48.9,38.1 48.9,36.2 | 48.9,36.2 D7.1 50.7,36.35 52.83,38.48 57.78,38.48 58.83,39.52 J7.3 | D3.2 48.9,36.2
  Bottom 2.032: v57.78,22.86 57.78,25.02 51.44,31.37 48.01,31.37 46.99,32.38 TP4.T 46.99,36.2 v48.9,38.1
N$1
  Top 0.203: Q1.1 7.37,27.56 8.26,26.67 8.26,26.11 8.53,25.83 10.59,25.83 R13.1 R1.1
N$2
  Top 0.203: 20.95,37.67 U6.16 20.94,38.5 20.7,38.73 19.94,38.73 19.68,38.48 19.68,36.45 19.43,36.2 19.43,33.4 18.29,32.26 R12.2
N$3  (via drill 0.3 pad 0.64)
  Top 0.203: R6.1 v15.11,35.43
  Bottom 0.406: J9.7 15.15,35.39 v15.11,35.43
N$4
  Top 0.203: R11.2 19.05,29.97 19.05,32.38 19.94,33.27 19.94,36.07 20.29,36.41 U6.15 20.22,37.72
N$5
  Top 0.406: R2.2 LED1.-
N$6
  Top 0.203: U6.19 22.89,38.56 22.62,38.83 21.86,38.83 21.59,38.56 U6.17 21.59,36.32 C12.2
N$7
  Top 0.254: R3.2 PWR.+
N$8
  Top 0.406: R14.2 LED2.+
N$9
  Top 0.406: R15.2 LED3.-
N$10
  Top 0.406: R16.2 LED4.+
N$11  (via drill 0.3 pad 0.64)
  Top 0.203: R20.2 R25.2 15.49,33.91 14.37,35.04 14.37,36.2 15.11,36.94 v15.11,37.59
  Bottom 0.406: J9.5 v15.11,37.59
N$12  (via drill 0.3 pad 0.64)
  Top 0.203: R23.1 R21.2 17.14,44.83 13.21,40.89 v13.21,40.77
  Bottom 0.254: J9.3 14.18,39.79 v13.21,40.77
N$13  (via drill 0.3)
  Top 0.203: R24.1 20.45,46.23 18.16,46.23 17.91,45.97 R22.2 17.14,43.81 v14.22,40.89
  Bottom 0.203: J9.2 v14.23,40.89 v14.22,40.89
N$14
  Top 0.203: U2.P$7 41.02,18.41 39.95,17.34 39.95,13.9 42.47,11.38 49.26,11.38 R17.8
N$15
  Top 0.203: R17.7 50.55,11.63 50.39,11.79 42.67,11.79 40.37,14.09 40.37,16.67 40.84,17.14 U2.P$8
N$16
  Top 0.203: R17.6 51.31,11.68 50.8,12.19 42.88,12.19 40.81,14.25 40.81,15.63 41.03,15.85 42.14,15.85 U2.P$9
N$17
  Top 0.254: R4.2 20.3,4.72 21.08,3.94 RST.+
N$21
  Top 0.203: R18.3 arc-90 61.85,13.59
  Top 0.305: U2.P$13 57.86,17.14 61.42,13.59 61.85,13.59 62.05,13.59
N$22
  Top 0.203: R18.2 61.9,14.35 61.85,14.35
  Top 0.305: U2.P$14 57.4,18.41 61.47,14.35 61.85,14.35 62.05,14.35
N$23
  Top 0.203: R18.1 61.98,15.24
  Top 0.305: 62.09,15.24 61.98,15.24 61.33,15.24 57.65,18.92 57.28,18.92 56.64,19.56 55.63,19.56 U2.P$15
N$31
  Top 0.203: RX.+ 31.75,36.32 31.75,40.51 R9.1
N$32
  Top 0.203: R10.1 TX.+
P5V
  Top 1.016: Q1.2 7.24,24.13 F1.1
PB0  (via drill 0.3 pad 0.64)
  Top 0.203: U1.9 41.48,50.8 38.98,48.3 37.51,48.3 36.98,47.77 36.98,34.56 34.33,31.9 24.18,31.9 21.13,28.85 21.13,18.9 23.12,16.91 U4.12 25.64,16.91 v25.65,16.89 | U5.2 50.55,7.37 50.67,7.49 50.67,8.38 50.42,8.64 49.91,8.64 49.72,8.83 R17.1 49.72,9.46 49.67,9.46 49.38,9.75 48.77,9.75 48.05,10.47 47.05,10.47 45.72,9.14 42.27,9.14 36.17,15.24 36.17,16.36 v35.55,16.98
  Bottom 0.203: v25.65,16.89 35.46,16.89 v35.55,16.98
PB1
  Top 0.203: U1.10 36.58,48.26 36.58,34.73 34.16,32.31 23.98,32.31 20.73,29.06 20.73,18.49 23.16,16.05 24.34,16.05 | 24.38,16.05 24.34,16.05 | 24.34,16.05 U4.13
PB2
  Top 0.203: U4.14 23.3,15.31 20.33,18.28 20.33,18.3 20.32,18.32 20.32,29.27 23.76,32.72 33.97,32.72 36.17,34.91 36.17,50.39 U1.11
PB3/MOSI  (via drill 0.3, 0.3 pad 0.64)
  Top 0.203: R21.1 18.67,43.81 18.92,43.56 21.97,43.56 v22.35,43.18 | v64.55,16.05 64.5,16 61.34,16 60.96,16.38 v60.96,18.29 | v25.55,14.73 25.33,14.51 U4.15 23.46,14.51 19.88,18.1 19.88,29.41 23.59,33.12 33.76,33.12 35.69,35.05 35.69,47.05 v35.36,47.38 34.04,48.7 U1.12 | v37.06,13.21 37.58,13.21 42.05,8.74 46.43,8.74 v47.47,9.78
  Bottom 0.203: v22.35,43.18 22.61,42.93 29.52,42.93 33.97,47.38 v35.36,47.38 | 26.03,15.21 v25.55,14.73 | v37.06,13.21 37.08,13.18 37.08,12.83 36.31,12.05 30.81,12.05 29.4,13.46 29.4,14.68 28.88,15.21 26.03,15.21 | 26.03,15.21
  Bottom 0.254: U1.32 64.77,26.67 64.77,24.38 63.25,22.86 63.25,17.36 v64.55,16.05 | v60.96,18.29 60.96,13.93 57.19,10.16 47.85,10.16 v47.47,9.78
PB4/MISO  (via drill 0.3, 0.3 pad 0.64)
  Top 0.203: R6.2 18.67,38.48 18.67,39.6 19.91,40.84 29.57,40.84 v29.9,40.51 | v37.52,12.32 37.87,12.32 41.86,8.33 47.5,8.33 v48.36,9.2 | v26.57,14.49 26.05,13.97 25.4,13.97 25.14,13.71 U4.16 23.48,13.71 19.45,17.73 19.45,29.61 23.37,33.53 33.54,33.53 34.92,34.91 34.92,34.92 35.22,35.22 35.22,39.51 v34.92,39.8 35.25,40.13 35.25,46.44 31.5,50.19 U1.13
  Bottom 0.203: 36.51,11.62 30.6,11.62 28.96,13.27 28.96,14.37 28.59,14.73 26.81,14.73 v26.57,14.49 | 36.51,11.62 | 36.51,11.62 36.82,11.62 v37.52,12.32 | v29.9,40.51 34.21,40.51 v34.92,39.8
  Bottom 0.254: U1.36 61.72,28.7 61.72,13.95 57.42,9.65 48.82,9.65 v48.36,9.2
PB5/SCK  (via drill 0.3, 0.3 pad 0.64)
  Top 0.203: 25.77,13.18 25.79,13.2 25.79,13.21 v25.82,13.23 25.82,12.26 U4.17 | v20.46,31.56 20.79,31.56 23.16,33.93 33.31,33.93 34.51,35.13 v34.51,38.73 34.23,39.01 34.23,40.13 34.84,40.74 34.84,46.14 31.64,49.34 30.42,49.34 U1.14 | R20.1 19.18,37.47 19.18,39.5 20.12,40.44 28.96,40.44 v29.9,39.5 | v37.86,11.37 38.21,11.37 41.66,7.92 47.75,7.92 48.36,8.53 v49.02,8.53
  Bottom 0.203: v20.46,31.56 20.12,31.22 20.12,17.04 23.95,13.21 25.8,13.21 v25.82,13.23 28.36,13.23 30.42,11.18 37.67,11.18 v37.86,11.37 | v29.9,39.5 33.74,39.5 v34.51,38.73
  Bottom 0.254: U1.35 62.23,26.67 62.23,13.76 57.61,9.14 49.63,9.14 v49.02,8.53
PC0  (via drill 0.3 pad 0.64)
  Top 0.203: U1.17 50.8,3.45 50.39,3.86 47.95,3.86 46.74,5.08 39.42,5.08 33.33,11.18 30.89,11.18 30.57,11.49 U4.23 30.57,13.72 29.67,14.63 v29.67,15.44 | v2.44,42.67 2.44,37.57 4.06,35.94 5.92,35.94 J4.1
  Bottom 0.203: v29.67,15.44 29.45,15.66 22.84,15.66 20.93,17.57 20.93,30.07 25.4,34.54 25.4,39.62 24.18,40.84 19.71,40.84 17.68,42.88 8.08,42.88 6.35,41.15 3.96,41.15 v2.44,42.67 2.44,51.33 TP8.T
PC1  (via drill 0.3 pad 0.64)
  Top 0.203: U1.18 51.61,4.27 48.16,4.27 46.94,5.49 39.62,5.49 32.89,12.22 U4.24 31.38,13.53 30.48,14.43 30.48,15.93 v30.28,16.13 | v3.45,42.67 3.45,38.71 4.19,37.97 5.95,37.97 J4.2
  Bottom 0.203: v30.28,16.13 22.96,16.13 21.34,17.75 21.34,29.87 25.81,34.34 25.81,39.83 24.38,41.25 19.91,41.25 17.88,43.28 7.72,43.28 6.1,41.66 4.47,41.66 v3.45,42.67 3.45,49.81 TP9.T
PC2
  Top 0.203: U9.3 36.17,29.27 36.17,27.43 33.73,24.99 33.73,21.54 31.86,19.67 31.86,13.86 32.01,13.71 U4.25 33.84,13.71 34.14,13.41 34.14,11.62 39.86,5.89 47.14,5.89 48.36,4.67 53.75,4.67 U1.19
PC3
  Top 0.203: U4.26 33.85,14.51 34.54,13.81 34.54,11.85 40.09,6.3 47.35,6.3 48.56,5.08 55.88,5.08 U1.20
  Top 0.254: C22.2 R19.1 59.05,8.38 60.18,7.25 J2.2
  Bottom 0.254: J2.2 61.09,7.24 61.09,5.21 U1.20
PC4/SDA
  Top 0.203: U4.27 33.92,15.31 34.95,14.28 34.95,12.07 40.31,6.71 47.55,6.71 48.77,5.49 58.01,5.49 U1.21
PC5/SCL
  Top 0.203: U4.28 34.06,16.11 35.36,14.81 35.36,12.24 40.48,7.11 47.75,7.11 48.97,5.89 60.15,5.89 U1.22
PD0/RX  (via drill 0.3 pad 0.64)
  Top 0.203: U4.30 34.37,17.71 34.95,18.29 34.95,24.38 38.2,27.64 38.2,30.89 40.51,33.2 40.51,40.48 41.5,41.47 v41.5,44.27 41.5,46.18 42.27,46.94 49.52,46.94 v49.78,46.67 | v33.21,44.68 32.92,44.68 R7.2
  Bottom 0.203: v49.78,46.67 56.96,46.67 59.69,49.4 62.1,49.4 U1.1 | v33.21,44.68 41.1,44.68 v41.5,44.27
PD1/TX  (via drill 0.3 pad 0.64)
  Top 0.203: U4.31 34.16,18.51 34.54,18.9 34.54,24.59 37.8,27.84 37.8,31.09 40.07,33.36 40.07,40.66 41.05,41.64 41.05,43.36 v40.77,43.64 40.77,46.05 42.06,47.35 50.39,47.35 v51.05,48.01 | R8.2 v33.27,43.18
  Bottom 0.203: v51.05,48.01 57.53,48.01 59.69,50.16 60.33,50.16 U1.2 | v33.27,43.18 38.3,43.18 38.81,43.69 40.72,43.69 v40.77,43.64
PD2/INT0  (via drill 0.3 pad 0.64)
  Top 0.203: U4.32 33.74,19.31 34.14,19.71 34.14,24.79 37.39,28.04 37.39,31.29 39.62,33.53 39.62,41.25 v39.83,41.45 40.53,42.16 40.53,42.89 40.01,43.42 40.01,46.1 41.66,47.75 49.66,47.75 50.67,48.77 56.39,48.77 U1.3 | J5.1 v10.16,44.02
  Bottom 0.203: v39.83,41.45 39.62,41.66 20.12,41.66 17.88,43.89 10.29,43.89 v10.16,44.02 10.16,48.9 TP6.T
PD3/INT1  (via drill 0.3 pad 0.64)
  Top 0.203: U4.1 31.77,20.8 33.33,22.35 33.33,25.2 35.15,27.03 35.15,29.7 39.12,33.67 39.12,41.76 v39.83,42.47 39.83,42.93 39.52,43.23 39.52,46.26 41.43,48.16 49.43,48.16 50.48,49.21 54.29,49.21 U1.4 | v11.38,44.7 11.43,44.7 11.94,44.2 11.94,40.26 11.67,39.99 J5.2
  Bottom 0.203: v39.83,42.47 39.42,42.06 20.32,42.06 17.67,44.71 11.39,44.71 | 11.39,44.71 v11.38,44.7 | 11.39,44.71 11.39,50.21 TP7.T
PD4  (via drill 0.3, 0.3 pad 0.64)
  Top 0.203: U4.2 30.57,21.63 30.89,21.95 32.31,21.95 32.92,22.55 32.92,25.4 34.75,27.23 34.75,29.95 38.67,33.87 38.67,42.51 v38.94,42.77 38.94,46.35 41.15,48.56 49.2,48.56 50.29,49.66 52.2,49.66 U1.5 | v21.4,42.86 18.48,42.86 R22.1
  Bottom 0.203: 21.34,42.93 v21.4,42.86 21.77,42.49 38.66,42.49 v38.94,42.77
PD5  (via drill 0.3 pad 0.64)
  Top 0.203: U1.6 48.97,48.97 40.86,48.97 38.23,46.34 38.23,34.03 34.88,30.68 24.79,30.68 22.35,28.25 22.35,19.91 22.96,19.31 U4.9 v26.16,19.31 v26.16,19.3 | R17.2 50.55,9.91 50.29,10.16 48.97,10.16 48.21,10.92 46.88,10.92 45.52,9.55 42.47,9.55 36.58,15.44 v36.58,18.92
  Bottom 0.203: v36.58,18.92 26.54,18.92 v26.16,19.3
PD6  (via drill 0.3 pad 0.64)
  Top 0.203: U1.7 46.84,49.38 40.64,49.38 37.8,46.53 37.8,34.19 34.69,31.09 24.59,31.09 21.95,28.45 21.95,19.71 23.15,18.51 U4.10 25.56,18.51 v25.65,18.41 | 63.32,14.4 R18.7 62.79,14.4 62.61,14.22 62.61,12.32 62.36,12.06 61.09,12.06 60.83,12.32 60.83,13.14 v59.54,14.44 | v44.5,10.71 42.53,10.71 38.2,15.04 v38.2,15.44
  Bottom 0.203: v25.65,18.41 35.84,18.41 38.2,16.05 v38.2,15.44 | v44.5,10.71 45.17,11.38 57.1,11.38 58.8,13.08 58.8,14.19 59.04,14.43 59.52,14.43 v59.54,14.44
PD7  (via drill 0.3, 0.3 pad 0.64)
  Top 0.203: U8.2 64.51,14.63 64.26,14.38 64.26,13.72 | 64.14,13.59 63.48,13.59 R18.6 63.17,13.64 | 64.26,13.72 64.14,13.59 | 64.26,13.72 64.26,13.46 | 64.26,13.46 64.26,12.57 63.25,11.56 60.98,11.56 60.35,12.19 60.35,12.69 v59.52,13.51 | v26.16,17.65 26.11,17.71 U4.11 23.13,17.71 21.54,19.3 21.54,28.65 24.38,31.5 34.5,31.5 37.37,34.36 37.39,34.39 37.39,47.21 v37.67,47.48 | v37.29,15.85 37.29,15.34 42.67,9.96 44.81,9.96 v45.52,10.67 | 64.14,13.59 64.26,13.46
  Bottom 0.203: U1.8 42.41,47.48 v37.67,47.48 | v26.16,17.65 35.99,17.65 37.29,16.36 v37.29,15.85 | v45.52,10.67 45.58,10.73 57.09,10.73 59.52,13.17 v59.52,13.51
RESET  (via drill 0.3 pad 0.64)
  Top 0.203: v19.71,32.11 19.71,32.46 22,34.75 32.91,34.75 33.37,35.21 33.37,40.48 33.96,41.07 33.96,45.69 33.53,46.13 31.98,46.13 31.75,46.35 31.75,47.67 31.06,48.36 22.55,48.36 C9.1 19.3,49.58 19.3,48.36 18.9,47.95 16.65,47.95 15.94,47.24 11.56,47.24 11.43,47.37 | U4.29 34.12,16.91 35.76,15.26 35.76,12.44 40.68,7.52 48.32,7.52 v48.51,7.71 | RESET.2 RESET.3 | RESET.3 11.11,47.2 11.18,47.14 11.18,47.31 RESET.3 | RESET.3 11.43,47.37 | 11.43,47.37 11.82,47.37
  Top 0.254: v47.37,2.54 47.37,1.65 46.74,1.02 34.54,1.02 U1.28 33.02,3.37 29.78,6.6 23.62,6.6 | RST.- 22.35,2.41 23.37,3.43 23.37,5.46 | 23.37,5.71 23.37,5.97 | 23.37,5.97 23.37,6.35 | 23.37,6.35 23.37,6.6 | 23.37,6.6 23.37,6.86 | 23.37,6.86 23.37,8.13 22.86,8.64 20.95,8.64 20.45,9.14 20.45,12.1 v21.49,13.14 | 23.37,5.71 23.11,5.71 | 23.11,5.71 22.35,5.71 R5.2 | 23.37,5.71 23.37,5.46 | 23.37,5.97 23.11,5.71 | 23.11,5.71 23.37,5.46 | 23.62,6.6 23.37,6.6 | 23.62,6.6 23.37,6.86 | 23.62,6.6 23.37,6.35
  Bottom 0.203: v19.71,32.11 19.71,16.87 21.49,15.09 v21.49,13.14
  Bottom 0.254: U1.34 62.74,24.64 62.74,13.59 57.78,8.64 50.24,8.64 49.31,7.71 v48.51,7.71 47.37,6.57 v47.37,2.54
USB_DM
  Top 0.203: J8.2 5.79,25.29 5.91,25.4 5.91,30.42 6.79,31.3 13.78,31.3 14.22,30.86 14.86,30.86 D10.2 16.64,30.73 R12.1
USB_DP
  Top 0.203: J8.3 5.91,24.64 6.35,25.07 6.35,30.23 6.99,30.86 13.6,30.86 13.97,30.49 13.97,29.21 14.22,28.96 D10.1 16.51,28.96 R11.1
VCC_3V3  (via drill 0.3 pad 0.64)
  Top 0.406: C27.2 15.37,38.99 v15.11,38.73
  Top 0.61: v23.37,11.18 26.26,8.28 30.94,8.28 35.56,3.66 U1.27
  Top 0.813: U3.2 v15.88,24.77 U3.4 16.89,24.77 17.02,24.64 v17.02,20.83 C13.2 17.02,18.73 C17.+
  Bottom 0.406: v15.88,26.67 15.88,27.94 12.9,30.91 12.9,37.42 14.21,38.73 v15.11,38.73 16.21,38.73 J9.4
  Bottom 0.61: v17.02,20.83 16.26,20.07 16.26,12.19 17.27,11.18 v23.37,11.18
  other vias: 17.78,26.67 17.78,24.77 17.78,22.86 15.88,22.86
  pour Top (isolate 0.254, no thermals): 15.11,27.3 18.92,27.3 18.92,22.23 15.11,22.23
  pour Bottom (isolate 0.254, no thermals): 13.34,27.3 18.92,27.3 18.92,22.23 13.34,22.23
VCC_5V  (via drill 0.3 pad 0.64)
  Top 0.203: R10.2 30.86,39.5
  Top 0.406: U4.6 27.38,19.87 | 27.38,19.87 27.69,19.56 | 27.69,19.56 28.7,19.56 28.96,19.81 28.96,20.78 U4.4 28.98,22.12 C5.2 C19.2 C25.1 30.35,28.54 U9.1 | C11.2 26.57,10.64 U4.18 26.57,12.96 27.38,13.76 27.38,19.87 | U2.P$12 57.28,15.88 C23.1 57.91,15.37 57.91,15.24 58.73,14.43 58.73,10.49 | C21.2 65.28,13.73 U8.5 | U5.5 53.23,8.02 C24.1 | 27.69,19.56 27.43,19.3 | 30.86,39.24 R10.2 R9.2 30.86,41.4 25.27,41.4 | 21.77,14.2 21.84,14.12 21.82,14.1 21.08,14.1 | 24.77,41.4 15.88,41.4 12.45,37.97 10.18,37.97 J5.3 | 24.77,41.4 25.02,41.4 | 25.02,41.4 25.27,41.4 | v25.02,43.59 25.02,41.66 | 25.02,41.66 25.02,41.4 | U6.4 26.79,45.86 26.29,46.35 C18.2 v27.05,46.99 C26.1 | 25.02,41.66 24.77,41.4 | 25.02,41.66 25.27,41.4 | 58.73,10.46 58.73,10.03 | R5.1 R4.1 | R4.1 R3.1 18.29,7.24 | R4.1 20.3,8.15 19.81,8.64 19.81,12.83 21.08,14.1 | 58.73,10.49 58.73,10.46 | 58.73,10.46 58.42,10.16 | 58.73,10.49 59.05,10.16 | 21.08,14.1 21.34,14.35 21.46,14.35 21.6,14.48 | 21.08,14.1 21.08,14.86
  Top 0.61: C21.2 65.28,12.57 v64.64,11.94 62.74,10.03 61.15,10.03 | C24.1 53.59,9.27 54.36,10.03 C28.1 | C11.2 26.62,10.49 26.62,9.75 27.1,9.27 31.37,9.27 U1.26 | 56.9,9.91 56.77,10.03 C28.1 | C28.1 58.73,10.03 61.07,10.03 | 5.99,40.01 J4.3 7.83,39.99 8.26,39.56 v8.26,37.97 10.14,37.97 J5.3 | 61.07,10.03 61.09,10.03 | 61.09,10.03 61.15,10.03 | 61.07,10.03 61.07,10.02 61.09,10.03 | J2.1 61.08,9.96 61.15,10.03
  Top 0.813: 13.34,18.16 13.78,18.16 C3.+ 13.91,17.91 | 13.34,18.16 U7.2 | F1.2 C4.+ C1.2 v12.32,21.34 C14.2 | C14.2 C20.2 13.21,18.29 13.34,18.16 | U3.3 13.59,23.24 13.21,22.86 C14.2 | 13.91,17.91 14.48,17.91 15.88,16.51 19.57,16.51 21.6,14.48 25.54,10.54 C11.2 | 13.72,17.91 13.91,17.91
  Bottom 0.406: v64.64,11.94 67.44,14.73 67.44,29.08 U1.31 | v25.02,43.59 25.02,45.97 26.04,46.99 v27.05,46.99
  Bottom 0.61: U1.26 39.5,1.14 47.75,1.14 48.39,1.78 48.39,5.71 50.42,7.75 57.94,7.75 59.46,9.27 61.06,9.27 J2.1 | v12.32,21.34 11.25,22.4 11.25,37.25 10.53,37.97 v8.26,37.97
VCC_12V  (via drill 0.3 pad 0.64, 1.02 pad 2.54)
  Top 0.61: 43.69,44.91 43.48,45.11 43.7,45.11 D5.1 | J1.+ 8.76,1.91
  Top 1.016: D3.1 D2.1 40.28,31.75 v39.62,31.09 39.62,27.78 35.82,23.98 35.82,21.9 38.04,19.68 38.73,19.68 | U2.P$6 39.75,19.68 | 39.75,19.68 38.73,19.68 | D4.1 43.72,42.27 | 43.72,42.27 43.72,44.88 43.69,44.91 | v42.47,42.27 43.28,42.27 | 43.28,42.27 43.72,42.27 | 43.28,42.27 43.69,42.67 | 43.28,42.27 43.69,41.86 | v38.76,18.52 38.76,18.69 | 38.76,18.96 38.76,19.66 38.73,19.68 | 38.76,18.69 38.76,18.96 | 38.76,18.96 37.97,19.75 | 38.76,18.69 39.75,19.68
  Top 3.048: v15.88,5.08 13.46,5.08 13.46,4.95 13.34,4.83 | 8.76,1.91 11.98,1.91 13.34,3.25 13.34,4.83 | 13.34,4.83 D1.2
  Bottom 1.016: v39.62,31.09 39.62,38.61 42.47,41.45 v42.47,42.27
  Bottom 3.048: v38.76,18.52 40.29,16.99 40.29,10.71 38.47,8.89 19.68,8.89 v15.88,5.08
  pour Top (isolate 0.254, no thermals): 14.63,3.66 11.94,3.66 11.94,6.71 14.63,6.71
VCC_USB  (via drill 0.3 pad 0.64)
  Top 0.254: v4.83,26.54 J8.1
  Top 0.406: R13.2 10.67,27.56 11.94,28.83 13.41,28.83 14.3,27.94 18.61,27.94 v18.73,28.07 | U6.20 23.54,36.53 v24.55,35.52 25.36,35.52 C2.1
  Top 0.61: Q1.3 9.27,26.92 | 9.27,26.92 v9.27,27.94 9.27,28.96 C10.2 | 9.27,26.92 10.16,26.92 R13.2
  Bottom 0.406: v18.73,28.07 18.8,28.13 18.8,32.4 20.74,34.35 23.38,34.35 v24.55,35.52
  Bottom 0.61: v9.27,27.94 6.22,27.94 v4.83,26.54
  pour Top (isolate 0.254, no thermals): 4.06,26.92 5.59,26.92 5.59,25.78 4.06,25.78
VIN  (via drill 0.3 pad 0.64)
  Top 0.61: v17.55,12.22 17.3,12.22 16.26,11.18 C15.+ | U1.23 44.2,4.06 38,4.06 31.65,10.41 30.24,10.41 v29.63,11.02
  Top 1.016: C15.+ 16.26,10.29 14.95,8.98 D1.1 C16.2 11.81,11.3 11.05,12.06 11.05,13.46 U7.1
  Bottom 0.61: v17.55,12.22 17.58,12.19 28.46,12.19 v29.63,11.02
XTAL1
  Top 0.305: U4.7 26.57,22.89 C6.2 27.18,25.02 X1.2
XTAL2
  Top 0.305: U4.8 25.77,22.61 C8.2 24.89,25.02 X1.1

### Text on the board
tPlace: JP1 | JP2 | - | M1 | + | - | M2 | + | JP3 | JP4
bPlace: TX | RX | D9 | D8 | D7 | D6 | D5 | D4 | D3 | D2 | D1 | D0 | GND | D13 | D12 | D11 | D10 | AREF | M1+ | M1- | M2- | M2+ | V1.2 08/28/2013 | SPI | MISO | VCC | VCC | GND | SIG | SCK | MOSI | RST | GND | WARNING / HOT SURFACE | RST | 3V3 | 5V | GND | GND | VIN | A0 | A1 | A2 | A3 | A4 | A5 | VCC_12V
